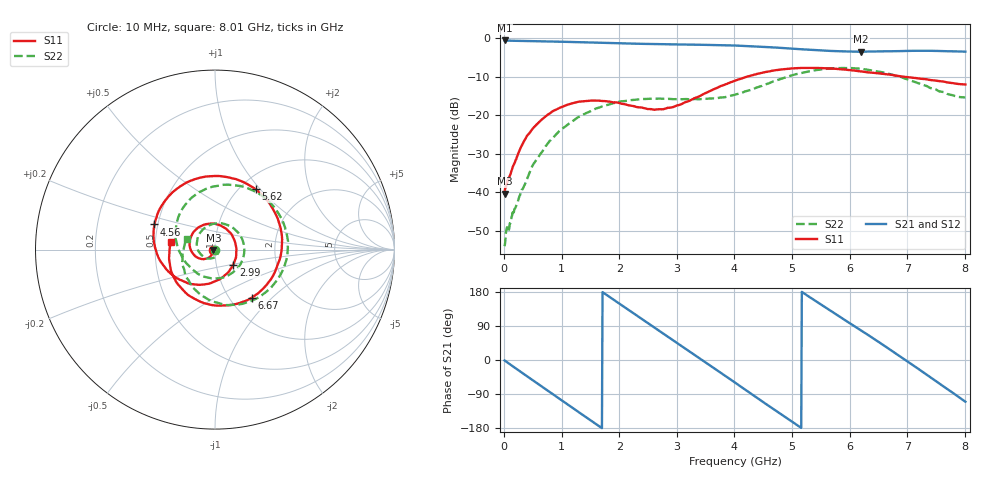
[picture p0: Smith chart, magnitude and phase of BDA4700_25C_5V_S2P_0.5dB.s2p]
!Agilent Technologies,E5071B,MY42404982,A.09.10
!Date: Mon Oct 20 13:26:12 2025
!Data & Calibration Information:
!Freq	S11:SOLT2(ON)	S21:SOLT2(ON)	S12:SOLT2(ON)	S22:SOLT2(ON)
# Hz S RI R 50
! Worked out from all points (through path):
!   801 points, 10 MHz to 8.01 GHz, reference 50 ohm
!   highest |S21| = -0.62 dB at 10 MHz (marker M1); lowest = -3.5 dB at 6.2 GHz (marker M2)
!   group delay of S21, straight-line fit = 286 ps
!   lowest |S11| = -40.4 dB at 10 MHz (marker M3), VSWR 1.02, Z = 49.1 - j0.241 ohm
!   |S11| at or under -10 dB: start of sweep to 4.218 GHz; 6.923 GHz to end of sweep
!   |S22| runs from -54.0 to -7.8 dB; largest |S21 - S12| = 0.0071
!   S11 on the Smith chart (normalised r, x): 10 MHz: 0.98, -0.00; 2.99 GHz: 1.21, -0.21; 4.56 GHz: 0.48, +0.15; 5.62 GHz: 1.17, +0.94; 6.67 GHz: 1.26, -0.76; 8.01 GHz: 0.60, +0.05
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1e7  -0.00928 -0.00246  0.9308 -0.0198  0.9308 -0.0208  -0.0019 -0.000633
3.6e8  -0.0274 -0.0391  0.7147 -0.5726  0.7145 -0.573  0.0123 -0.00235
7.2e8  -0.0818 -0.0508  0.2065 -0.8811  0.2063 -0.8814  0.00278 -0.0392
1.02e9  -0.1286 -0.0138  -0.2833 -0.8488  -0.2836 -0.8493  -0.0483 -0.0474
1.35e9  -0.1377 0.0612  -0.7064 -0.5287  -0.7068 -0.5294  -0.0991 0.0108
1.63e9  -0.0972 0.1202  -0.8638 -0.1135  -0.8642 -0.1133  -0.0851 0.0906
1.92e9  -0.0232 0.1451  -0.7925 0.3321  -0.7927 0.3325  -0.004 0.1443
2.32e9  0.0772 0.1007  -0.3691 0.7591  -0.3691 0.7594  0.1292 0.0944
2.68e9  0.1189 0.00836  0.1614 0.8189  0.1617 0.819  0.1593 -0.0386
2.99e9  0.1014 -0.0855  0.5663 0.603  0.5656 0.6026  0.093 -0.1314
3.49e9  -0.0321 -0.1894  0.8132 -0.073  0.8133 -0.0736  -0.0674 -0.148
4.01e9  -0.2451 -0.1352  0.4047 -0.6895  0.4057 -0.6891  -0.1766 -0.0526
4.56e9  -0.3372 0.1401  -0.3522 -0.6797  -0.3524 -0.6803  -0.2156 0.1332
4.96e9  -0.1988 0.3484  -0.6831 -0.2638  -0.6842 -0.266  -0.1144 0.3016
5.35e9  0.0524 0.4062  -0.6659 0.2217  -0.667 0.2199  0.1128 0.3575
5.62e9  0.2259 0.3358  -0.4822 0.4845  -0.4822 0.486  0.2777 0.2881
6.2e9  0.3691 -0.0167  0.139 0.6502  0.1452 0.6513  0.3908 -0.0799
6.67e9  0.2065 -0.2669  0.5789 0.3447  0.5796 0.3439  0.184 -0.2916
6.68e9  0.2011 -0.2704  0.5849 0.3335  0.5864 0.3332  0.1784 -0.2939
7.24e9  -0.1177 -0.2722  0.6026 -0.325  0.6017 -0.3256  -0.1044 -0.2293
7.63e9  -0.2438 -0.1229  0.2348 -0.6354  0.234 -0.6367  -0.1829 -0.0801
8.01e9  -0.247 0.0404  -0.2296 -0.6254  -0.2282 -0.6264  -0.1585 0.061
